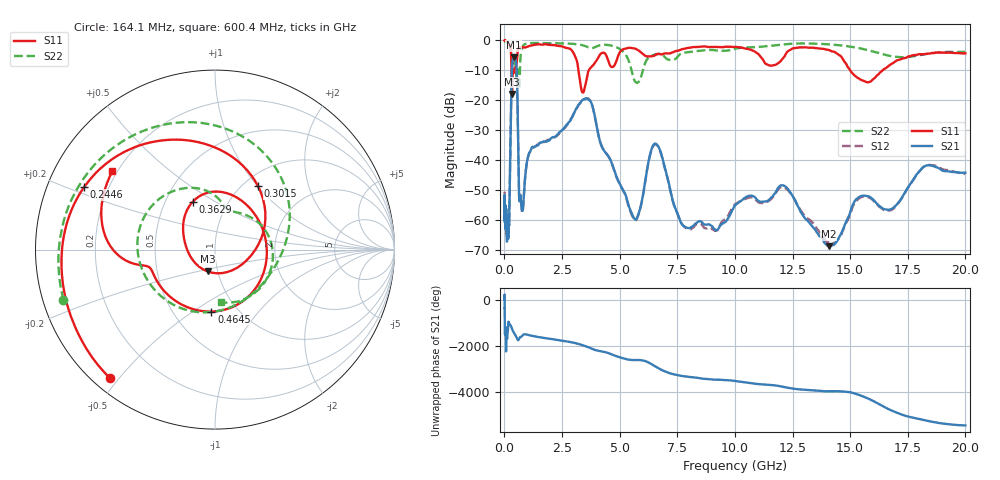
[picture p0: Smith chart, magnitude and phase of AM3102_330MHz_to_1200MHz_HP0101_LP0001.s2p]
! Date/Time: Tue, Sep 11, 2018 5:13 PM
! Network Analyzer: Agilent Technologies E8362B Rev: A.07.50.63
! Sweep from 0.010 to 20.000 GHz, 1601 Points, Sweep Type: LOG
! Power Supply: 4.949 V, 0.001 A
# Hz S DB R 50
!freq MagS11 AngS11 MagS21 AngS21 MagS12 AngS12 MagS22 AngS22
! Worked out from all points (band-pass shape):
!   1601 points, 10 MHz to 20 GHz, reference 50 ohm
!   highest |S21| = -5.66 dB at 414.5 MHz (marker M1); lowest = -68.7 dB at 14.07 GHz (marker M2)
!   |S21| within 3 dB of the highest: 333.1 MHz to 525.3 MHz (192.2 MHz wide, 44.8 % of centre)
!   lowest |S11| = -17.8 dB at 331.5 MHz (marker M3), VSWR 1.29, Z = 44.7 - j11.1 ohm
!   |S11| at or under -10 dB: 309.7 MHz to 370.5 MHz (60.84 MHz wide, 17.9 % of centre); 3.211 GHz to 3.66 GHz (448.5 MHz wide, 13.1 % of centre); 15.01 GHz to 16.4 GHz (1.399 GHz wide, 8.91 % of centre)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
!   |S22| runs from -16.2 to -0.2 dB; largest |S21 - S12| = 0.0068
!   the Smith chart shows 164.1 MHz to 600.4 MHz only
!   S11 on the Smith chart (normalised r, x): 164.1 MHz: 0.05, -0.47; 244.6 MHz: 0.11, +0.23; 301.5 MHz: 1.16, +1.01; 362.9 MHz: 0.69, +0.40; 464.5 MHz: 0.76, -0.60; 600.4 MHz: 0.18, +0.33
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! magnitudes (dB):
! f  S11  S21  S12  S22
! 10 MHz  0.0  -53.3  -54.1  -0.2
! 35.55 MHz  0.0  -58.2  -58.8  -0.4
! 126.4 MHz  -0.4  -64.7  -63.0  -0.8
! 164.1 MHz  -0.7  -65.5  -63.7  -1.0
! 244.6 MHz  -1.9  -43.3  -43.5  -2.0
! 301.5 MHz  -7.4  -17.2  -17.2  -4.8
! 331.5 MHz  -17.8  -8.9  -8.9  -8.7
! 362.9 MHz  -10.6  -6.4  -6.5  -9.5
! 414.5 MHz  -10.8  -5.7  -5.7  -7.5
! 447.2 MHz  -9.7  -5.9  -5.9  -7.2
! 464.5 MHz  -9.2  -6.0  -6.1  -7.5
! 538.2 MHz  -7.4  -10.6  -10.7  -12.6
! 600.4 MHz  -2.9  -35.1  -35.1  -10.6
! 776 MHz  -2.3  -56.9  -57.4  -2.2
! 1.59 GHz  -1.4  -34.0  -34.1  -0.8
! 3.634 GHz  -10.5  -19.6  -19.4  -2.3
! 5.652 GHz  -2.7  -59.6  -60.1  -13.5
! 6.58 GHz  -4.7  -34.5  -34.7  -4.6
! 7.882 GHz  -2.6  -62.5  -62.7  -4.0
! 12.09 GHz  -5.9  -48.4  -49.0  -1.3
! 14.07 GHz  -3.2  -68.7  -67.5  -1.3
! 20 GHz  -4.3  -44.2  -44.6  -3.8
